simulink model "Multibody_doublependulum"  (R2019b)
settings: Solver=VariableStepAuto  StartTime=0.0  StopTime=10.0  MaxStep=0.01  RelTol=1e-3
undefined symbols (not defined in the file): deg, kg, m, N, s, X, Y, Z
libraries: sm_lib x7, nesl_utility x2

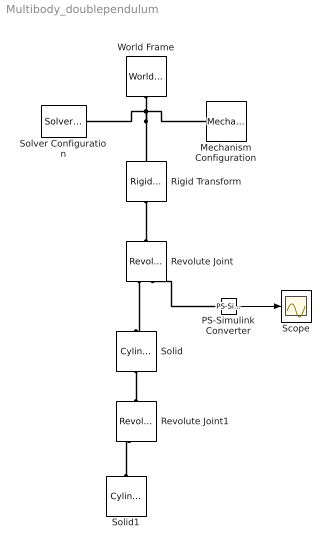
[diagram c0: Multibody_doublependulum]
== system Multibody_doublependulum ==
  Mechanism Configuration : sm_lib/Utilities/Mechanism Configuration  UniformGravity=Constant  GravityVector=[0 0 -9.80665]  GravityUnits=m/s^2  LinearizationDelta=0.001
  PS-Simulink Converter : nesl_utility/PS-Simulink Converter  PhysicalDomain=network_engine_domain  SubClassName=ps_output  LeftPortType=input  RightPortType=output  PseudoPeriodic=off  Frequencies=[]  Unit=deg  AffineConversion=off
  Revolute Joint : sm_lib/Joints/Revolute Joint  JointMode=Normal  SenseConstraintForce=off  SenseConstraintForceX=off  SenseConstraintForceY=off  SenseConstraintForceZ=off  SenseConstraintTorque=off  SenseConstraintTorqueX=off  SenseConstraintTorqueY=off  SenseConstraintTorqueZ=off  SenseTotalForce=off  SenseTotalForceX=off  SenseTotalForceY=off  SenseTotalForceZ=off  SenseTotalTorque=off  SenseTotalTorqueX=off  SenseTotalTorqueY=off  SenseTotalTorqueZ=off  CompositeWrenchDir=FollowerOnBase  CompositeWrenchFrame=BaseFrame  EquilibriumPosition=0  EquilibriumPositionUnits=deg  SpringStiffness=0  SpringStiffnessUnits=N*m/deg  DampingCoefficient=0  DampingCoefficientUnits=N*m/(deg/s)  TorqueActuationMode=NoTorque  MotionActuationMode=ComputedMotion  SensePosition=on  SenseVelocity=off  SenseAcceleration=off  SenseTorqueForce=off  SenseLowerLimitTorqueForce=off  SenseUpperLimitTorqueForce=off  LowerLimitSpecify=off  LowerLimitBound=-90  LowerLimitBoundUnits=deg  LowerLimitStiffness=1e4  LowerLimitStiffnessUnits=N*m/deg  LowerLimitDamping=10  LowerLimitDampingUnits=N*m/(deg/s)  LowerLimitTransitionRegionWidth=0.1  LowerLimitTransitionRegionWidthUnits=deg  UpperLimitSpecify=off  UpperLimitBound=90  UpperLimitBoundUnits=deg  UpperLimitStiffness=1e4  UpperLimitStiffnessUnits=N*m/deg  UpperLimitDamping=10  UpperLimitDampingUnits=N*m/(deg/s)  UpperLimitTransitionRegionWidth=0.1  UpperLimitTransitionRegionWidthUnits=deg  PositionTargetSpecify=on  PositionTargetPriority=High  PositionTargetValue=45  PositionTargetValueUnits=deg  VelocityTargetSpecify=off  VelocityTargetPriority=High  VelocityTargetValue=0  VelocityTargetValueUnits=deg/s
  Revolute Joint1 : sm_lib/Joints/Revolute Joint  JointMode=Normal  SenseConstraintForce=off  SenseConstraintForceX=off  SenseConstraintForceY=off  SenseConstraintForceZ=off  SenseConstraintTorque=off  SenseConstraintTorqueX=off  SenseConstraintTorqueY=off  SenseConstraintTorqueZ=off  SenseTotalForce=off  SenseTotalForceX=off  SenseTotalForceY=off  SenseTotalForceZ=off  SenseTotalTorque=off  SenseTotalTorqueX=off  SenseTotalTorqueY=off  SenseTotalTorqueZ=off  CompositeWrenchDir=FollowerOnBase  CompositeWrenchFrame=BaseFrame  EquilibriumPosition=0  EquilibriumPositionUnits=deg  SpringStiffness=0  SpringStiffnessUnits=N*m/deg  DampingCoefficient=0  DampingCoefficientUnits=N*m/(deg/s)  TorqueActuationMode=NoTorque  MotionActuationMode=ComputedMotion  SensePosition=on  SenseVelocity=off  SenseAcceleration=off  SenseTorqueForce=off  SenseLowerLimitTorqueForce=off  SenseUpperLimitTorqueForce=off  LowerLimitSpecify=off  LowerLimitBound=-90  LowerLimitBoundUnits=deg  LowerLimitStiffness=1e4  LowerLimitStiffnessUnits=N*m/deg  LowerLimitDamping=10  LowerLimitDampingUnits=N*m/(deg/s)  LowerLimitTransitionRegionWidth=0.1  LowerLimitTransitionRegionWidthUnits=deg  UpperLimitSpecify=off  UpperLimitBound=90  UpperLimitBoundUnits=deg  UpperLimitStiffness=1e4  UpperLimitStiffnessUnits=N*m/deg  UpperLimitDamping=10  UpperLimitDampingUnits=N*m/(deg/s)  UpperLimitTransitionRegionWidth=0.1  UpperLimitTransitionRegionWidthUnits=deg  PositionTargetSpecify=on  PositionTargetPriority=High  PositionTargetValue=45  PositionTargetValueUnits=deg  VelocityTargetSpecify=off  VelocityTargetPriority=High  VelocityTargetValue=0  VelocityTargetValueUnits=deg/s
  Rigid Transform : sm_lib/Frames and Transforms/Rigid Transform  TranslationMethod=None  TranslationStandardOffset=0  TranslationLengthUnit=m  TranslationStandardAxis=+Z  TranslationCartesianOffset=[0 0 0]  TranslationROffset=0  TranslationROffsetUnits=m  TranslationZOffset=0  TranslationZOffsetUnits=m  TranslationThetaOffset=0  TranslationThetaOffsetUnits=deg  RotationMethod=StandardAxis  RotationAngleUnits=deg  RotationStandardAxis=+X  RotationAngle=-90  RotationArbitraryAxis=[0 0 1]  FollAlignAxisA=+X  BaseAlignAxisA=+Y  FollAlignAxisB=+Y  BaseAlignAxisB=+Z  RotationSequenceAxes=FollowerAxes  RotationSequence=XYX  RotationSequenceAngles=[0 0 0]  RotationSequenceAnglesUnits=deg  RotationMatrix=[1 0 0; 0 1 0; 0 0 1]
  Scope : Scope
  Solid : sm_lib/Body Elements/Cylindrical Solid  GraphicAmbientColor=[0.15 0.15 0.15 1.0]  BasedOnType=Density  CenterOfMass=[0 0 0]  CenterOfMassUnits=m  GraphicDiffuseColor=[0.4 0.4 1.0]  CylinderLength=1  CylinderLengthUnits=m  CylinderRadius=0.02  CylinderRadiusUnits=m  Density=7850  DensityUnits=kg/m^3  DoExposeReferenceFrame=off  GraphicEmissiveColor=[0.0 0.0 0.0 1.0]  ExportEntireGeometry=off  SerializedFrames=<Frames><Frame><Id>Frame1</Id><Value><Name>F1</Name><Origin><Source>GeometricFeature</Source><FeatureName>top curve</FeatureName></Origin><PrimaryAxis><DefinedDirection>+Z</DefinedDirection><Source>ReferenceFrame</Source><SourceDirection>+Y</SourceDirection><FeatureName></FeatureName></PrimaryAxis><SecondaryAxis><DefinedDirection>+X</DefinedDirection><Source>ReferenceFrame</Source><SourceDirection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  MarkerShape=Sphere  MarkerSize=10  GraphicType=FromGeometry  InertiaType=CalculateFromGeometry  Mass=1  MassUnits=kg  MomentsOfInertia=[1 1 1]  MomentsOfInertiaUnits=kg*m^2  GraphicOpacity=1.0  ProductsOfInertia=[0 0 0]  ProductsOfInertiaUnits=kg*m^2  GraphicShininess=75  GraphicSpecularColor=[0.5 0.5 0.5 1.0]  GraphicVisPropType=SimpleVisualProperties
  Solid1 : sm_lib/Body Elements/Cylindrical Solid  GraphicAmbientColor=[0.15 0.15 0.15 1.0]  BasedOnType=Density  CenterOfMass=[0 0 0]  CenterOfMassUnits=m  GraphicDiffuseColor=[0.4 0.4 1.0]  CylinderLength=1  CylinderLengthUnits=m  CylinderRadius=0.02  CylinderRadiusUnits=m  Density=7850  DensityUnits=kg/m^3  DoExposeReferenceFrame=off  GraphicEmissiveColor=[0.0 0.0 0.0 1.0]  ExportEntireGeometry=off  SerializedFrames=<Frames><Frame><Id>Frame1</Id><Value><Name>F1</Name><Origin><Source>GeometricFeature</Source><FeatureName>top curve</FeatureName></Origin><PrimaryAxis><DefinedDirection>+Z</DefinedDirection><Source>ReferenceFrame</Source><SourceDirection>+Y</SourceDirection><FeatureName></FeatureName></PrimaryAxis><SecondaryAxis><DefinedDirection>+X</DefinedDirection><Source>ReferenceFrame</Source><SourceDirection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  MarkerShape=Sphere  MarkerSize=10  GraphicType=FromGeometry  InertiaType=CalculateFromGeometry  Mass=1  MassUnits=kg  MomentsOfInertia=[1 1 1]  MomentsOfInertiaUnits=kg*m^2  GraphicOpacity=1.0  ProductsOfInertia=[0 0 0]  ProductsOfInertiaUnits=kg*m^2  GraphicShininess=75  GraphicSpecularColor=[0.5 0.5 0.5 1.0]  GraphicVisPropType=SimpleVisualProperties
  Solver Configuration : nesl_utility/Solver Configuration  PhysicalDomain=network_engine_domain  SubClassName=solver  LeftPortType=input  RightPortType=generic  Tones=[]  Harmonics=[]  SimulateNoise=off  Profile=off  UseLocalSampling=off  EnableSwitchedLinearOptims=on  FrequencyDomain=off  UseCCode=off  RelTol=0.001  AbsTol=1e-06  MinStep=1e-09  ToWorkspace=off  RevertToSquareIcSolve=off  NumHomotopyIterations=100  PhasorMode=off  PhasorModeNumHarmonics=1  DoDC=off  ResidualTolerance=1e-09  UseLocalSolver=off  LocalSolverChoice=NE_BACKWARD_EULER_ADVANCER  LocalSolverSampleTime=0.001  DoFixedCost=off  MaxNonlinIter=3  MaxModeIter=2  LinearAlgebra=auto  EquationFormulation=NE_TIME_EF  DelaysMemoryBudget=1024  AutomaticFiltering=on  FilteringTimeConstant=0.001  PartitionStorageMethod=AS_NEEDED  PartitionMemoryBudget=1024  PartitionMethod=FAST
  World Frame : sm_lib/Frames and Transforms/World Frame
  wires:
  PS-Simulink Converter/1 -> Scope/1
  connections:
  World Frame/RConn1 -- Rigid Transform/LConn1 -- Mechanism Configuration/RConn1 -- Solver Configuration/RConn1
  Revolute Joint/RConn1 -- Solid/LConn1
  Revolute Joint/LConn1 -- Rigid Transform/RConn1
  PS-Simulink Converter/LConn1 -- Revolute Joint/RConn2
  Revolute Joint1/LConn1 -- Solid/RConn1
  Solid1/LConn1 -- Revolute Joint1/RConn1
